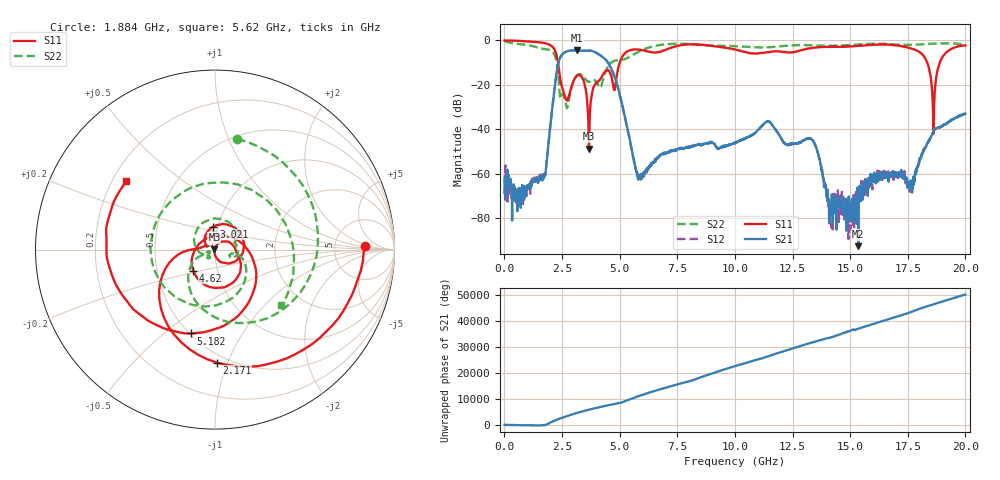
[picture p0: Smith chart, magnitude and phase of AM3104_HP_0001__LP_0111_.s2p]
!Created with skrf (http://scikit-rf.org).
# Hz S RI R 50.0
!freq ReS11 ImS11 ReS21 ImS21 ReS12 ImS12 ReS22 ImS22
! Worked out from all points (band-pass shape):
!   1601 points, 10 MHz to 20 GHz, reference 50 ohm
!   highest |S21| = -4.40 dB at 3.146 GHz (marker M1); lowest = -92.8 dB at 15.35 GHz (marker M2)
!   |S21| within 3 dB of the highest: 2.437 GHz to 4.256 GHz (1.819 GHz wide, 54.4 % of centre)
!   lowest |S11| = -48.8 dB at 3.671 GHz (marker M3), VSWR 1.01, Z = 49.7 + j0.213 ohm
!   |S11| at or under -10 dB: 2.325 GHz to 5.002 GHz (2.678 GHz wide, 73.1 % of centre); 18.34 GHz to 18.89 GHz (542.6 MHz wide, 2.92 % of centre)
!   |S22| runs from -30.5 to -0.2 dB; largest |S21 - S12| = 0.005
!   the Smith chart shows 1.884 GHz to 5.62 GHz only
!   S11 on the Smith chart (normalised r, x): 1.884 GHz: 11, +2; 2.171 GHz: 0.44, -0.91; 3.021 GHz: 0.95, +0.25; 4.62 GHz: 0.76, -0.18; 5.182 GHz: 0.51, -0.62; 5.62 GHz: 0.26, +0.32
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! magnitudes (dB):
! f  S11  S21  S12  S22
! 10 MHz  0.0  -68.7  -60.9  -0.2
! 659.7 MHz  -0.2  -70.7  -72.5  -1.6
! 1.884 GHz  -1.6  -49.5  -49.3  -4.0
! 2.171 GHz  -4.0  -22.0  -22.0  -6.4
! 2.684 GHz  -26.7  -5.0  -5.0  -29.3
! 3.021 GHz  -17.8  -4.5  -4.5  -17.8
! 3.146 GHz  -15.9  -4.4  -4.4  -15.7
! 3.346 GHz  -16.2  -4.6  -4.6  -15.5
! 3.671 GHz  -48.8  -4.7  -4.6  -18.6
! 4.62 GHz  -15.5  -12.4  -12.3  -10.1
! 5.182 GHz  -6.3  -32.3  -32.3  -8.5
! 5.62 GHz  -4.1  -54.0  -54.4  -6.3
! 6.682 GHz  -5.2  -52.4  -52.4  -2.1
! 10.01 GHz  -4.0  -46.1  -46.0  -2.6
! 13.34 GHz  -3.3  -44.6  -44.6  -2.2
! 14.17 GHz  -2.9  -73.8  -76.5  -2.3
! 15.35 GHz  -2.5  -92.8  -75.1  -1.8
! 16.68 GHz  -1.9  -61.5  -61.2  -1.6
! 17.66 GHz  -3.6  -66.5  -67.9  -1.9
! 18.61 GHz  -42.1  -41.0  -40.8  -1.4
! 19.01 GHz  -7.3  -38.4  -38.5  -1.3
! 20 GHz  -2.2  -33.1  -32.9  -1.7
